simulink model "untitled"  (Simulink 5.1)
settings: Solver=ode45  StartTime=0.0  StopTime=10.0  RelTol=1e-3
undefined symbols (not defined in the file or in its folder): data, WriteDymolaHeader

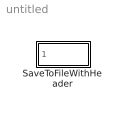
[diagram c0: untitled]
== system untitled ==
  SaveToFileWithHeader : Subsystem  InitFcn=WriteDymolaHeader;  StopFcn=|  mask(SaveToFile){Filename=data.mat}
      | Filename = get_param (gcb, 'Filename');                           
      | eval (['!copy /B untitled_header.mat + untitled.mat ' Filename ]);
      mask help: This blocks saves the data of the connected bus into a file. Additionally to the "ToFile" matlab block he also saves: - names and hierarchy of signals - description to signal (currently same as name) - position of signal (currently same position as in bus) Data is stored with given name in a mat-4-file. The file can be viewed easily with Dymola even for very big file sizes.

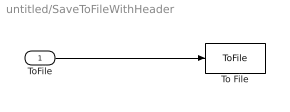
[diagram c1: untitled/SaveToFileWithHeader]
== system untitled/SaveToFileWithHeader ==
  ToFile : Inport
  To File : ToFile  MatrixName=data_2
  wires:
  ToFile/1 -> To File/1
